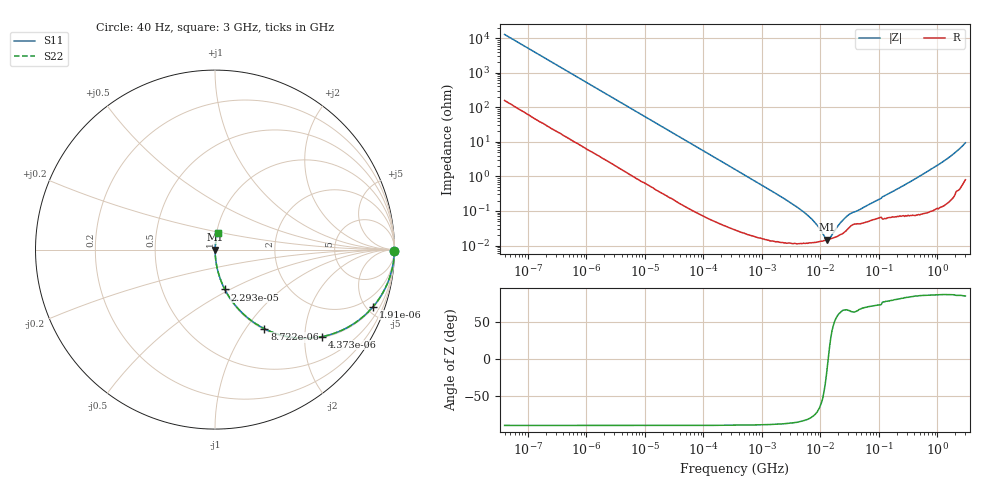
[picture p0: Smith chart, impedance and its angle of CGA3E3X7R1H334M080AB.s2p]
! S-parameter Generated by TDK Corporation
! Copyright(C) 2015 TDK Corporation.
! All Rights Reserved.
! TDK P/N: CGA3E3X7R1H334M080AB (Multilayer Ceramic Chip Capacitors)
! Property: C=330nF
! Size(LxWxT): 1.6x0.8x0.8mm, 0.063x0.031x0.031inches
! Model Type: s2p (Touchstone File Format Version 1.0)
! Frequency: DC=Yes Start=0.00004MHz Stop=3000MHz 396points Log-sweep
! Note: This model was converted from impedance.
! Model Generated on Jun. 23, 2015
! Hash(MD5):
! Port Assignments:
!  1 ---| |--- 2
! Applicable Conditions:
!  Temperature = 25 degC
!  DC Bias Voltage = 0 V
!  Small Signal Operation
! Terms and conditions regarding TDK Simulation Models
! (1)This simulation model is being provided solely for informational purposes. Please refer to the specifications of the products in terms of detailed characteristics of such products.
! (2)In no event shall TDK Corporation of any of its subsidiaries be liable for any loss or damage arising, directly or indirectly,
!  From any information contained in this simulation model, including, but not limited to loss or damages arising from any inaccuracies, omissions or errors in connection with such information.
! (3)Any and all copyrights on this simulation model are owned by TDK Corporation.
!  Duplication or redistribution of this simulation model without prior written permission from TDK Corporation is prohibited.
! (4)This simulation model is subject to any modification or change without any prior notice.
! (5)Neither TDK Corporation nor any of its subsidiaries shall make any warranty, express or implied,
!  Including but not limited to the correctness, implied warranties of merchantability and fitness for a particular purpose with respect to this simulation models.
! (6)The use of this simulation model shall be deemed to have consented to the terms and conditions hereof.
# MHz S MA R 50
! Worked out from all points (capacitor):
!   395 points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, 40 Hz to 3 GHz, reference 50 ohm
!   read as one part in series: C = 311 nF near 41.88 Hz
!   lowest |Z| = 14.9 mohm at 13.14 MHz (marker M1)
!   series resonance near 13.55 MHz, so ESL is about 440 pH
!   S11 on the Smith chart (normalised r, x): 40 Hz: open; 1.91 kHz: 1.07, -5.52; 4.373 kHz: 1.03, -2.43; 8.722 kHz: 1.01, -1.22; 22.93 kHz: 1.01, -0.47; 3 GHz: 1.02, +0.19
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4e-05  0.9999 -0.4  0.007826 88.8  0.007826 88.8  0.9999 -0.4
0.0002520917  0.9983 -2.8  0.04845 86.5  0.04845 86.5  0.9983 -2.8
0.000834128  0.9857 -9.0  0.1569 80.3  0.1569 80.3  0.9857 -9.0
0.001909884  0.9367 -19.8  0.3391 69.5  0.3391 69.5  0.9367 -19.8
0.002889976  0.8732 -28.5  0.4768 60.8  0.4768 60.8  0.8732 -28.5
0.00437302  0.7674 -39.2  0.6321 50.1  0.6321 50.1  0.7674 -39.2
0.008721545  0.5195 -58.0  0.8485 31.3  0.8485 31.3  0.5195 -58.0
0.01739424  0.2943 -72.2  0.9523 17.1  0.9523 17.1  0.2943 -72.2
0.0229261  0.2285 -76.1  0.9708 13.2  0.9708 13.2  0.2285 -76.1
0.06918777  0.07872 -84.8  0.9959 4.5  0.9959 4.5  0.07872 -84.8
0.3464102  0.01601 -88.1  0.9996 0.9  0.9996 0.9  0.01601 -88.1
2.877491  0.001872 -86.2  0.9999 0.1  0.9999 0.1  0.001872 -86.2
4.998775  0.0009779 -83.2  0.9999 0.1  0.9999 0.1  0.0009779 -83.2
7.22376  0.0005693 -77.7  0.9999 0.0  0.9999 0.0  0.0005693 -77.7
13.14015  0.0001487 -9.5  0.9999 0.0  0.9999 0.0  0.0001487 -9.5
14.40706  0.0001618 18.4  0.9998 -0.0  0.9998 -0.0  0.0001618 18.4
21.8003  0.0004511 62.7  0.9998 -0.0  0.9998 -0.0  0.0004511 62.7
30.08671  0.0007685 65.7  0.9997 -0.0  0.9997 -0.0  0.0007685 65.7
150.6385  0.003262 78.4  0.9993 -0.2  0.9993 -0.2  0.003262 78.4
1195.011  0.02553 85.6  0.9984 -1.5  0.9984 -1.5  0.02553 85.6
2173.747  0.05434 82.9  0.9947 -3.1  0.9947 -3.1  0.05434 82.9
3000  0.09255 79.8  0.9878 -5.3  0.9878 -5.3  0.09255 79.8
